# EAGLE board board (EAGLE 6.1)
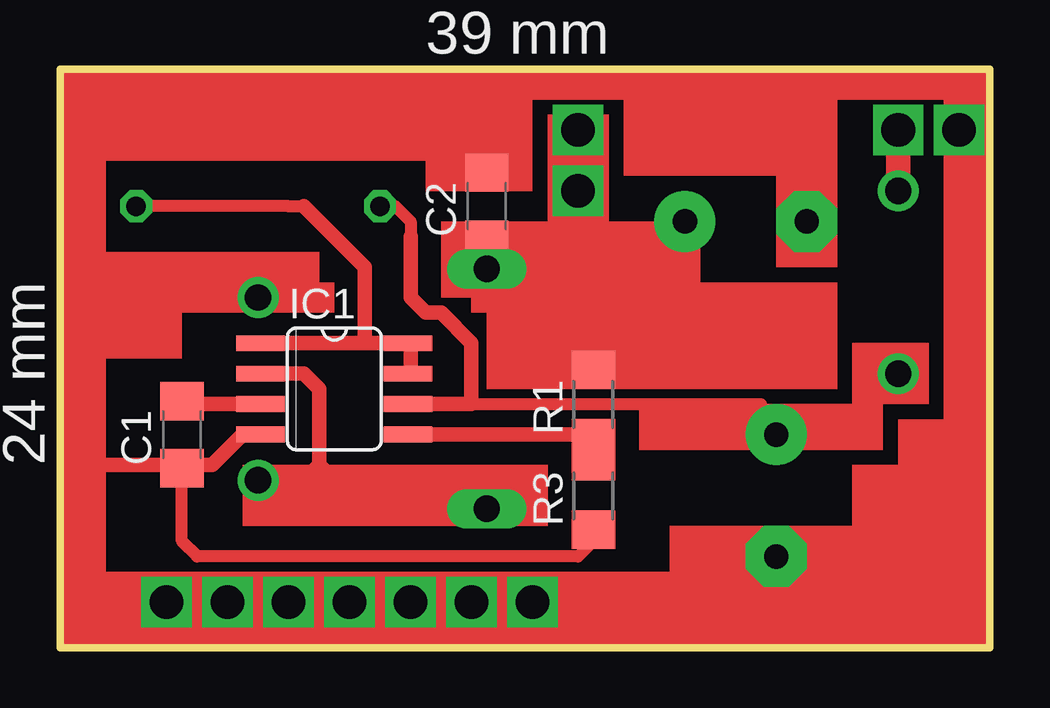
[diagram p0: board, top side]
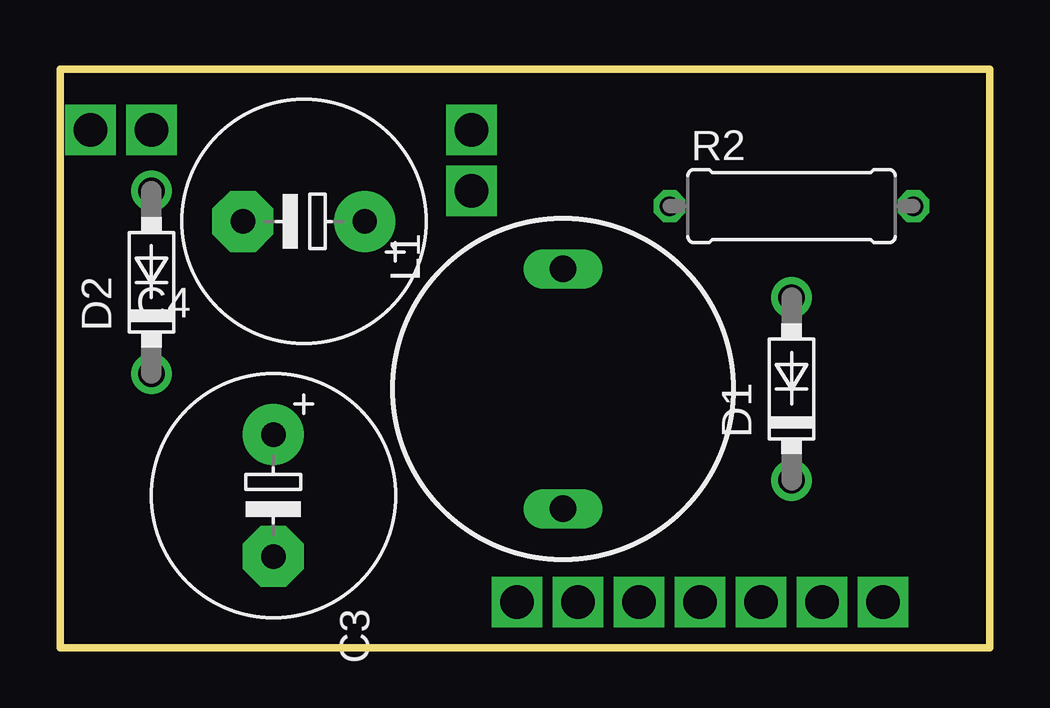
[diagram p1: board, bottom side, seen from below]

Size 38.73 x 24.13 mm. Coordinates in mm from the lower left corner, seen from the top.
Outline: 0,24.13 38.73,24.13 38.73,0 0,0 0,24.13
Copper layers (1*16): Top 0.035mm / dielectric 1.5mm / Bottom 0.035mm
Design rules: minimum track width 10mil, minimum drill 24mil, track to track 8mil, track to pad 8mil, pad to pad 8mil, via to via 8mil, smd to smd 8mil, copper to edge 40mil, drill to drill 8mil, minimum pad ring 10mil, minimum via ring 8mil, stop-mask expansion 4mil, vias tented up to drill 0mil, thermal gap 10mil

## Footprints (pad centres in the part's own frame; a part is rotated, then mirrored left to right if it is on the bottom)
C1206 = smd 1.6 x 1.8: 1 -1.4,0; 2 1.4,0
E5-10,5 = drill 1.016 pad 2.54: + -2.54,0 | drill 1.016 pad 2.54 octagon: - 2.54,0
DO41-7.6 = drill 1.1 pad 1.7: A 3.81,0; C -3.81,0
SO08 = smd 0.66 x 2.032: 1 -1.905,-3.073; 2 -0.635,-3.073; 3 0.635,-3.073; 4 1.905,-3.073; 5 1.905,3.073; 6 0.635,3.073; 7 -0.635,3.073; 8 -1.905,3.073
SD14 = drill 1.1 long: 1 -5,0; 2 5,0
R1206 = smd 1.6 x 1.803: 1 -1.422,0; 2 1.422,0
0309/10 = drill 0.813 octagon: 1 -5.08,0; 2 5.08,0

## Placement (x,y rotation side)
C1  [C1206]  5.08,8.89 90 top
C2  [C1206]  17.78,18.41 90 top
C3  [E5-10,5]  29.84,6.35 270 bottom
C4  [E5-10,5]  28.57,17.78 180 bottom
D1  [DO41-7.6]  8.26,10.8 90 bottom
D2  [DO41-7.6]  34.93,15.24 90 bottom
IC1  [SO08]  11.43,10.8 270 top
L1  [SD14]  17.78,10.8 90 bottom
R1  [R1206]  22.23,10.16 90 top
R2  [0309/10]  8.26,18.41 0 bottom
R3  [R1206]  22.23,6.35 90 top

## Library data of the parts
C1-C4 R1-R3 = rcl
D1 D2 = diode
IC1 = motorola-sensor-driver
L1 = inductor-neosid

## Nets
S$1: R2.2
S$2: D1.C
S$6: D1.A
S$19: D2.A
S$20: R2.1

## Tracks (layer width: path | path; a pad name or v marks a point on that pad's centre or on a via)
S$1
  Top 0.508: 10.16,18.41 9.52,18.41 R2.2
  Top 0.61: 8.26,12.7 12.7,12.7 | 12.7,12.7 14.6,12.7 14.6,11.43 | 12.7,12.7 12.7,15.88 10.16,18.41
S$2
  Top 0.61: 8.89,11.43 10.16,11.43 10.8,10.8 10.8,7.62 | 10.8,7.62 10.16,6.98 D1.C | 10.8,7.62 11.43,6.98 14.6,6.98 15.88,5.71 17.78,5.71
S$3
  Top 0.61: 5.08,10.16 8.26,10.16
S$4
  Top 0.61: 14.6,8.89 22.23,8.89
S$5
  Top 0.61: 8.26,8.89 7.62,8.89 6.35,7.62 1.27,7.62
S$6
  Top 0.61: D1.A 7.62,14.6
S$9
  Top 0.508: 22.23,4.45 21.59,3.81 5.71,3.81 5.08,4.45 5.08,6.98
S$10  (via drill 1.4 pad 0.81)
  Top 1.016: 33.02,3.81 37.46,8.26 v37.46,21.59 37.46,23.49 2.54,23.49 1.27,22.23 1.27,20.32
S$11  (via drill 1.4 pad 0.81)
  other vias: 4.45,1.91
S$12  (via drill 1.4 pad 0.81)
  other vias: 6.98,1.91
S$13  (via drill 1.4 pad 0.81)
  other vias: 9.52,1.91
S$14  (via drill 1.4 pad 0.81)
  other vias: 12.06,1.91
S$15  (via drill 1.4 pad 0.81)
  other vias: 14.6,1.91
S$16  (via drill 1.4 pad 0.81)
  other vias: 17.14,1.91
S$17  (via drill 1.4 pad 0.81)
  other vias: 19.69,1.91
S$18  (via drill 1.4 pad 0.81)
  Top 0.61: 22.23,12.06 v21.59,19.05
  Top 1.016: 17.78,15.88 20.32,15.88 21.59,17.14 21.59,17.78 v21.59,19.05 v21.59,21.59
S$19  (via drill 1.4 pad 0.81)
  Top 1.016: v34.93,21.59 D2.A
S$20
  Top 0.508: R2.1 13.97,18.41 14.6,17.78 14.6,17.14 | 17.14,10.16 29.21,10.16
  Top 0.61: 14.6,17.14 14.6,14.6 15.24,13.97 15.88,13.97 17.14,12.7 17.14,10.16 13.97,10.16
(copper drawn outside any net)
  shapes: Top area x31

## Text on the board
tNames: 39 mm | 24 mm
